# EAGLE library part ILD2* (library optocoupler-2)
Siemens ILD205/206/207/211/213/217 DUAL PHOTOTRANSISTOR SMALL OUTLINE SURFACE MOUNT OPTOCOUPLER Source: 153385-da-01-en-Optocoupler_ILD205-T.pdf
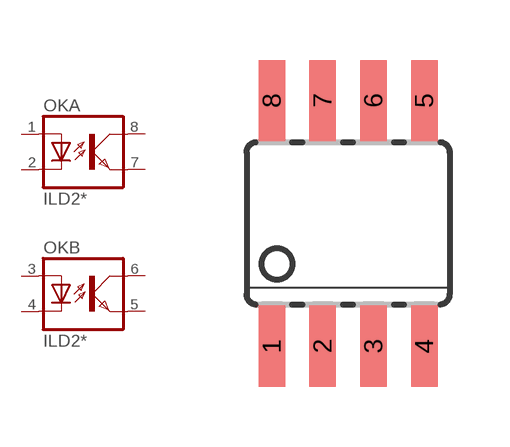
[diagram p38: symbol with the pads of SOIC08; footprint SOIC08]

Designator prefix OK; gates A=OK B=OK

## ILD205, ILD206, ILD207, ILD211, ILD213, ILD217  [SOIC08]
1  A:A  pas
2  A:C  pas
3  B:A  pas
4  B:C  pas
5  B:EMIT  pas
6  B:COL  pas
7  A:EMIT  pas
8  A:COL  pas

## Footprint SOIC08 (pad centres in mm)
Small Outline Package
smd 0.66 x 2.032: 1 -1.905,-3.073; 2 -0.635,-3.073; 3 0.635,-3.073; 4 1.905,-3.073; 5 1.905,3.073; 6 0.635,3.073; 7 -0.635,3.073; 8 -1.905,3.073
